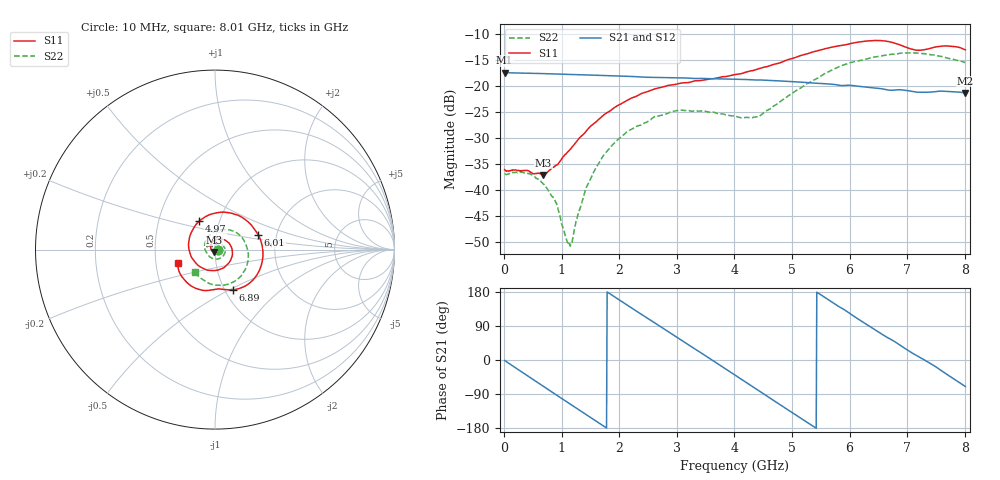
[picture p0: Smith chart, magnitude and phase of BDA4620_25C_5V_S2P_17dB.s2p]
!Agilent Technologies,E5071B,MY42404982,A.09.10
!Date: Wed May 06 09:01:52 2026
!Data & Calibration Information:
!Freq	S11:SOLT2(ON)	S21:SOLT2(ON)	S12:SOLT2(ON)	S22:SOLT2(ON)
# Hz S RI R 50
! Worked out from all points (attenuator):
!   801 points, 10 MHz to 8.01 GHz, reference 50 ohm
!   highest |S21| = -17.42 dB at 10 MHz (marker M1); lowest = -21.3 dB at 8.01 GHz (marker M2)
!   lowest |S11| = -37.1 dB at 680 MHz (marker M3), VSWR 1.03, Z = 49.6 - j1.35 ohm
!   |S11| at or under -10 dB: start of sweep to end of sweep
!   |S22| runs from -50.7 to -13.6 dB; largest |S21 - S12| = 0.00062
!   S11 on the Smith chart (normalised r, x): 10 MHz: 1.03, -0.00; 4.97 GHz: 0.80, +0.26; 6.01 GHz: 1.61, +0.28; 6.89 GHz: 1.09, -0.52; 8.01 GHz: 0.65, -0.11
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1e7  0.0157 -0.0011  0.1345 -0.00285  0.1347 -0.00291  0.0141 -0.000516
4.3e8  0.00825 -0.0129  0.0954 -0.092  0.0953 -0.0922  0.0134 -0.0055
6.8e8  -0.00341 -0.0136  0.0466 -0.1228  0.0465 -0.1231  0.00877 -0.00743
8.9e8  -0.0148 -0.0087  -0.000898 -0.1304  -0.00104 -0.1306  0.00325 -0.00715
1.13e9  -0.0233 0.00593  -0.0537 -0.1175  -0.0539 -0.1177  -0.00246 -0.00179
1.19e9  -0.0241 0.0107  -0.0655 -0.1109  -0.0658 -0.1112  -0.0034 0.000228
1.35e9  -0.0235 0.0237  -0.0931 -0.088  -0.0932 -0.0881  -0.005 0.00566
1.58e9  -0.0133 0.0424  -0.1188 -0.0443  -0.119 -0.0444  -0.00409 0.0153
1.87e9  0.0135 0.0577  -0.1239 0.0182  -0.1241 0.0184  0.00442 0.0262
2.68e9  0.0957 0.00062  -0.00372 0.1207  -0.00355 0.121  0.0478 0.0189
3.41e9  0.0337 -0.1075  0.111 0.0401  0.1113 0.0401  0.0442 -0.0366
4.01e9  -0.094 -0.0877  0.0893 -0.0744  0.0894 -0.0746  -0.0148 -0.0492
4.42e9  -0.1461 0.00757  0.0188 -0.1126  0.0187 -0.1127  -0.0498 -0.012
4.97e9  -0.0881 0.1585  -0.0787 -0.0773  -0.0788 -0.0774  -0.0371 0.074
5.35e9  0.0337 0.2085  -0.1061 -0.0128  -0.1062 -0.0127  0.0248 0.1084
6.01e9  0.2413 0.0818  -0.054 0.0861  -0.0541 0.0862  0.1558 0.0602
6.35e9  0.2634 -0.0649  0.0025 0.0965  0.00253 0.0966  0.1842 -0.0146
6.68e9  0.1825 -0.1941  0.0494 0.0768  0.0496 0.077  0.1739 -0.0974
6.89e9  0.1006 -0.2244  0.0728 0.0561  0.073 0.0563  0.1469 -0.1449
7.19e9  0.0189 -0.2188  0.0859 0.0142  0.0862 0.0143  0.0767 -0.1922
7.56e9  -0.0922 -0.2205  0.081 -0.037  0.0813 -0.037  -0.021 -0.1925
8.01e9  -0.2083 -0.0771  0.0293 -0.0806  0.0295 -0.0808  -0.1111 -0.1248
